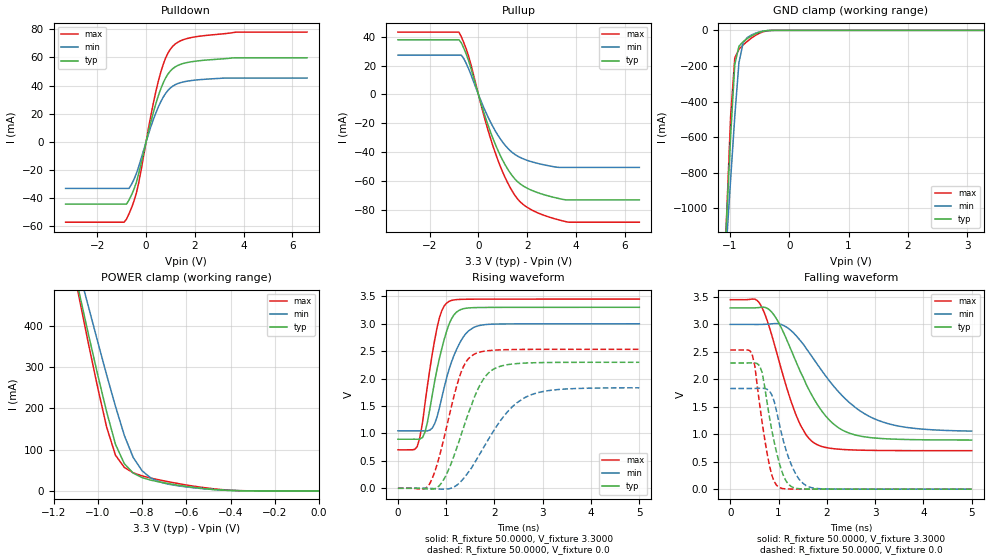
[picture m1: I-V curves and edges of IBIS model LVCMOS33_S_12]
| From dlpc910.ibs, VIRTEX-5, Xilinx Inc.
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|   Model GTL
|   Model LVCMOS33_S_12
[Model]  LVCMOS33_S_12
Model_type I/O
Polarity   Non-Inverting
Enable   Active-Low
Vinl = 0.76
Vinh = 2.2
Vmeas =  1.6500V
Cref =   0.0F
Rref =   1.0000M
Vref =   0.0V
C_comp   6.0000pF   6.0000pF   6.0000pF
[Model Spec]
Vinl   0.76   0.69   0.8
Vinh   2.2   2.0   2.3
[Temperature Range]   25.0000   85.0000   0.0
[Voltage Range]   3.3000V   3.0000V   3.4500V
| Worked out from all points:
|   slope of the pulldown table from 0 to 0.495 V, typ, clamps not added: 15.3 ohm
|   slope of the pullup table from 0 to 0.495 V, typ, clamps not added: 19 ohm
|   GND clamp passes 1 mA (typ) near -0.36 V on its own axis
|   POWER clamp passes 1 mA (typ) near -0.40 V on its own axis
|   rising waveform, R_fixture 50.0000, V_fixture 3.3000: 20-80 % time 346ps typ, 406ps min, 287ps max; typ from 0.894 V to 3.3 V
|   rising waveform, R_fixture 50.0000, V_fixture 0.0: 20-80 % time 568ps typ, 825ps min, 439ps max; typ from 0 V to 2.3 V
|   falling waveform, R_fixture 50.0000, V_fixture 3.3000: 20-80 % time 816ps typ, 1.12ns min, 583ps max; typ from 3.3 V to 0.895 V
|   falling waveform, R_fixture 50.0000, V_fixture 0.0: 20-80 % time 303ps typ, 358ps min, 256ps max; typ from 2.3 V to 0 V
[Pulldown]
|Voltage   I(typ)   I(min)   I(max)
-3.3V     -44.15mA   -33.01mA   -57mA
-900mV    -44.15mA   -33.01mA   -57mA
-800mV    -44.15mA   -33.01mA   -54.74mA
-700mV    -41.24mA   -33.01mA   -51.06mA
-400mV    -28.84mA   -22.58mA   -36.48mA
300mV     21.07mA    15.97mA    27.73mA
600mV     37.59mA    28.43mA    49.38mA
900mV     48.27mA    36.64mA    63.17mA
1.2V      53.36mA    40.7mA     69.61mA
1.9V      57.05mA    43.68mA    74.28mA
3.7V      59.71mA    45.39mA    78.01mA
6.6V      59.71mA    45.39mA    78.01mA
[Pullup]
|Voltage   I(typ)   I(min)   I(max)
-3.3V     37.94mA    27.29mA    43.29mA
-800mV    37.94mA    27.29mA    43.29mA
-700mV    35.83mA    27.29mA    40.04mA
-400mV    23.29mA    17.77mA    26.44mA
300mV     -16.58mA   -12.24mA   -19.33mA
800mV     -38.84mA   -28.33mA   -45.63mA
1.3V      -54.42mA   -38.99mA   -64.6mA
1.6V      -60.53mA   -42.79mA   -72.48mA
1.8V      -63.16mA   -44.46mA   -75.92mA
2.5V      -68.62mA   -48.18mA   -82.72mA
3.7V      -73.23mA   -50.68mA   -88.73mA
6.6V      -73.23mA   -50.68mA   -88.73mA
[GND_clamp]
|Voltage   I(typ)   I(min)   I(max)
-3.3V     -16.97A    -12.88A    -20.48A
-1.13V    -1.567A    -1.562A    -1.656A
-1.06V    -1.075A    -1.198A    -1.059A
-990mV    -594.4mA   -837.2mA   -482.9mA
-920mV    -191.9mA   -483.2mA   -155.6mA
-850mV    -89.88mA   -181.4mA   -105.9mA
-780mV    -63.96mA   -70.51mA   -82.33mA
-710mV    -46.62mA   -40.81mA   -61.99mA
-640mV    -31.71mA   -26.56mA   -43.7mA
-500mV    -9.786mA   -8.389mA   -15.42mA
-290mV    -155.5uA   -193.9uA   -401.9uA
3.28V     28.06nA    90.59uA    57.71nA
[POWER_clamp]
|Voltage   I(typ)   I(min)   I(max)
-3.28V    5.82A      5.011A     6.424A
-1.12V    567.4mA    604.5mA    564.7mA
-1.08V    470.7mA    523.2mA    456.9mA
-1.04V    374.3mA    442mA      351.1mA
-960mV    191.7mA    281.1mA    154.6mA
-920mV    112.8mA    204.8mA    86.55mA
-880mV    65.86mA    134.5mA    56.98mA
-840mV    43.25mA    81.04mA    43.8mA
-760mV    26.01mA    31.15mA    31.13mA
-680mV    17.61mA    16.23mA    22.15mA
-400mV    1.02mA     1.137mA    1.723mA
0V        29.68nA    137.7nA    65.13nA
[Ramp]
| variable   typ   min   max
dV/dt_r  1.3782/0.5667n   1.0992/0.8294n   1.5198/0.4365n
dV/dt_f  1.4431/0.8154n   1.1658/1.1227n   1.6493/0.5825n
R_load = 50.0000
[Rising Waveform]
R_fixture= 50.0000
V_fixture= 3.3000
V_fixture_min= 3.0000
V_fixture_max= 3.4500
|time   V(typ)   V(min)   V(max)
0s        894.1mV    1.047V     701mV
400ps     893.7mV    1.047V     762.7mV
560ps     1.024V     1.046V     1.543V
710ps     1.696V     1.096V     2.442V
810ps     2.171V     1.301V     2.926V
910ps     2.553V     1.657V     3.242V
1.06ns    2.995V     2.172V     3.408V
1.36ns    3.275V     2.766V     3.446V
1.67ns    3.296V     2.964V     3.448V
5ns       3.299V     2.999V     3.45V
[Rising Waveform]
R_fixture= 50.0000
V_fixture= 0.0
|time   V(typ)   V(min)   V(max)
0s        591nV      867.6nV    1.119uV
660ps     -16.07mV   -2.128mV   84.89mV
810ps     10.54mV    -11.47mV   429.9mV
1.01ns    262.6mV    -14.54mV   1.124V
1.31ns    975.6mV    129mV      2.12V
1.57ns    1.632V     441.2mV    2.441V
1.97ns    2.166V     1.031V     2.517V
2.32ns    2.26V      1.443V     2.529V
2.68ns    2.285V     1.676V     2.532V
5ns       2.297V     1.832V     2.533V
[Falling Waveform]
R_fixture= 50.0000
V_fixture= 3.3000
V_fixture_min= 3.0000
V_fixture_max= 3.4500
|time   V(typ)   V(min)   V(max)
0s        3.3V       3V         3.45V
610ps     3.309V     2.999V     3.382V
910ps     3.166V     3.014V     2.649V
1.36ns    2.325V     2.799V     1.356V
1.57ns    1.914V     2.566V     989.6mV
1.77ns    1.589V     2.315V     823.4mV
2.27ns    1.102V     1.747V     726.5mV
2.98ns    932.5mV    1.283V     705.7mV
3.69ns    903.6mV    1.12V      701.9mV
5ns       894.9mV    1.057V     701.2mV
[Falling Waveform]
R_fixture= 50.0000
V_fixture= 0.0
|time   V(typ)   V(min)   V(max)
0s        2.297V     1.833V     2.534V
450ps     2.3V       1.833V     2.468V
510ps     2.299V     1.833V     2.238V
660ps     2.124V     1.838V     1.217V
860ps     1.074V     1.719V     256.8mV
1.01ns    491mV      1.212V     33.03mV
1.16ns    141.7mV    698.5mV    4.93mV
1.31ns    28.68mV    355.2mV    2.03mV
1.62ns    2.534mV    44.23mV    959.3uV
5ns       29.51uV    86.48uV    37.28uV
